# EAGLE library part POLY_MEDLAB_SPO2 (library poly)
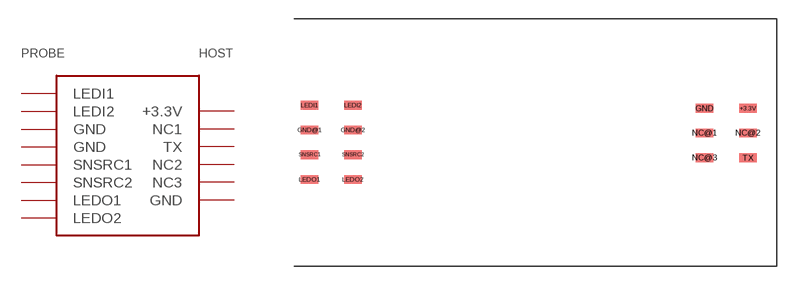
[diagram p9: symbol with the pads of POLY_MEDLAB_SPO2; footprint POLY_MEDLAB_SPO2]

Designator prefix -

## POLY_MEDLAB_SPO2  [POLY_MEDLAB_SPO2]
+3.3V  +3.3V
GND  GND  pwr
GND@1  GND  pwr
GND@2  GND  pwr
LEDI1  LEDI1  out
LEDI2  LEDI2  out
LEDO1  LEDO1  in
LEDO2  LEDO2  in
NC@1  NC1  nc
NC@2  NC2  nc
NC@3  NC3  nc
SNSRC1  SNSRC1
SNSRC2  SNSRC2
TX  TX

## Footprint POLY_MEDLAB_SPO2 (pad centres in mm)
smd 1.422 x 0.711: +3.3V 33.65,2.75; GND 30.15,2.75; GND@1 -1.75,1; GND@2 1.75,1; LEDI1 -1.75,3; LEDI2 1.75,3; LEDO1 -1.75,-3; LEDO2 1.75,-3; NC@1 30.15,0.75; NC@2 33.65,0.75; NC@3 30.15,-1.25; SNSRC1 -1.75,-1; SNSRC2 1.75,-1; TX 33.65,-1.25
